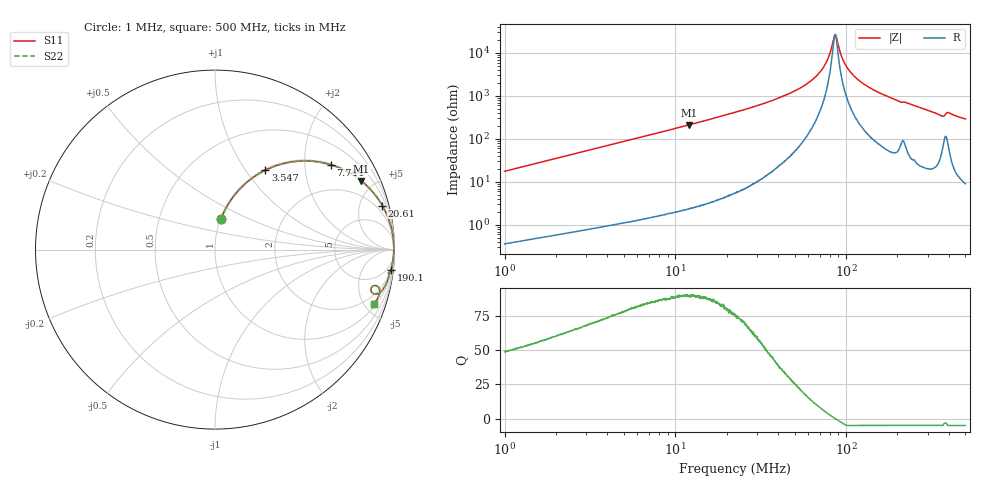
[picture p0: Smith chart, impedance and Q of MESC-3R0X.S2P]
!s-Parameter Generated by FASTRON Sdn. Bhd.
!FASTRON P/N : MESC-3R0X
!Keysight Technologies,E4991B,MY54100416,A.01.15
!Date: Mon Mar 16 10:46:10 2026
!Version  : Rev00 Mon Mar 16 10:46:10 2026
!Data & Calibration Information:
!PortZ  Port1:50+j0  Port2:50+j0
!When reading, reference impedance value at option line is always used.
! Remarks : This data is being provided solely for informational purposes.
!Freq	S11	S21	S12	S22
# Hz S dB R 50
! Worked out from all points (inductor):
!   1601 points, 1 MHz to 500 MHz, reference 50 ohm
!   read as one part in series: L = 2.8 uH near 1.032 MHz
!   highest Q = 90.3 at 12.01 MHz (marker M1), where L = 2.81 uH
!   self-resonance near 86.4 MHz
!   S11 on the Smith chart (normalised r, x): 1 MHz: 1.01, +0.35; 3.547 MHz: 1.02, +1.24; 7.744 MHz: 1.03, +2.71; 20.61 MHz: 1.10, +7.56; 190.1 MHz: 2, -17; 500 MHz: 1.18, -5.84
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1000000  -15.23 78.9  -0.16 -10.0  -0.16 -10.0  -15.23 78.9
2820919  -7.14 63.1  -1.00 -26.1  -1.00 -26.1  -7.14 63.1
3547441  -5.62 57.6  -1.46 -31.6  -1.46 -31.6  -5.62 57.6
7744141  -1.94 36.2  -4.57 -53.1  -4.57 -53.1  -1.94 36.2
7957584  -1.85 35.5  -4.73 -53.9  -4.73 -53.9  -1.85 35.5
1.201124e7  -0.91 25.1  -7.44 -64.2  -7.44 -64.2  -0.91 25.1
2.060919e7  -0.32 14.8  -11.87 -74.5  -11.87 -74.5  -0.32 14.8
2.236068e7  -0.27 13.5  -12.63 -75.7  -12.63 -75.7  -0.27 13.5
4.294146e7  -0.07 5.8  -19.98 -82.6  -19.98 -82.6  -0.07 5.8
6.307767e7  -0.04 2.4  -27.41 -83.2  -27.41 -83.2  -0.04 2.4
7.541731e7  -0.03 1.0  -34.68 -77.8  -34.68 -77.8  -0.03 1.0
8.47377e7  -0.03 0.1  -46.89 -35.2  -46.89 -35.2  -0.03 0.1
8.639945e7  -0.03 0.0  -48.65 -0.6  -48.65 -0.6  -0.03 0.0
8.843662e7  -0.03 -0.2  -46.25 38.8  -46.25 38.8  -0.03 -0.2
9.670074e7  -0.04 -0.9  -36.24 74.2  -36.24 74.2  -0.04 -0.9
1.086514e8  -0.04 -1.8  -30.21 80.5  -30.21 80.5  -0.04 -1.8
1.319406e8  -0.05 -3.3  -24.75 82.1  -24.75 82.1  -0.05 -3.3
1.77937e8  -0.10 -6.0  -19.59 80.8  -19.59 80.8  -0.10 -6.0
1.900828e8  -0.12 -6.7  -18.64 80.0  -18.64 80.0  -0.12 -6.7
3.580143e8  -0.58 -15.3  -11.50 68.4  -11.50 68.4  -0.58 -15.3
3.960579e8  -0.59 -13.0  -12.85 66.9  -12.85 66.9  -0.59 -13.0
5e8  -0.56 -18.7  -9.88 69.5  -9.88 69.5  -0.56 -18.7
